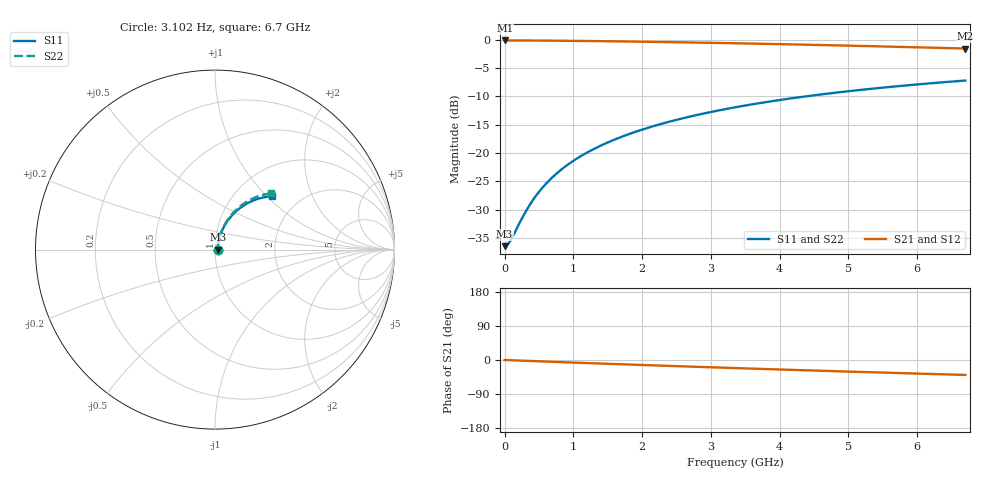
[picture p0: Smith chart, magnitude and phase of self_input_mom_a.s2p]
! Created Mon Jan 20 16:21:08 2014
# ghz S ma R 50
! 2 Port Network Data from data block
! freq  magS11  angS11  magS21  angS21  magS12  angS12  magS22  angS22
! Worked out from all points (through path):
!   107 points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, 3.102 Hz to 6.7 GHz, reference 50 ohm
!   highest |S21| = -0.13 dB at 3.102 MHz (marker M1); lowest = -1.6 dB at 6.7 GHz (marker M2)
!   group delay of S21, straight-line fit = 16.6 ps
!   lowest |S11| = -36.5 dB at 3.102 Hz (marker M3), VSWR 1.03, Z = 51.5 + j2.76e-08 ohm
!   |S11| at or under -10 dB: start of sweep to 4.386 GHz
!   |S22| runs from -36.5 to -7.1 dB; largest |S21 - S12| = 0
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3.101852e-09  0.01503 0.0  0.985 -0.0  0.985 -0.0  0.01503 0.0
0.003101852  0.01503 1.0  0.985 -0.0  0.985 -0.0  0.01503 1.0
0.03101852  0.01532 9.9  0.9849 -0.2  0.9849 -0.2  0.01529 9.9
0.06203704  0.01604 19.0  0.9849 -0.4  0.9849 -0.4  0.01602 19.0
0.09305556  0.01713 27.0  0.9848 -0.6  0.9848 -0.6  0.01712 27.1
0.2403935  0.02562 51.2  0.9843 -1.7  0.9843 -1.7  0.0256 51.3
0.3179398  0.03122 57.6  0.9839 -2.2  0.9839 -2.2  0.03118 57.7
0.4342593  0.04016 63.3  0.9831 -3.0  0.9831 -3.0  0.0401 63.4
0.5505787  0.04938 66.4  0.9821 -3.8  0.9821 -3.8  0.04932 66.6
0.6668981  0.05869 68.2  0.981 -4.6  0.981 -4.6  0.05865 68.5
0.7909722  0.06863 69.3  0.9796 -5.4  0.9796 -5.4  0.0686 69.6
0.9305556  0.07974 69.8  0.9779 -6.3  0.9779 -6.3  0.07973 70.3
1.116667  0.09439 70.0  0.9753 -7.5  0.9753 -7.5  0.09441 70.5
1.349306  0.1124 69.6  0.9717 -9.1  0.9717 -9.1  0.1124 70.2
1.628472  0.1334 68.7  0.967 -10.8  0.967 -10.8  0.1336 69.5
1.954167  0.1574 67.4  0.961 -12.9  0.961 -12.9  0.1576 68.3
2.303125  0.1823 65.8  0.954 -15.0  0.954 -15.0  0.1827 66.8
2.791667  0.216 63.3  0.9435 -18.0  0.9435 -18.0  0.2167 64.5
3.419792  0.2573 60.0  0.9286 -21.7  0.9286 -21.7  0.2585 61.4
4.466667  0.3209 54.4  0.9011 -27.6  0.9011 -27.6  0.3232 56.2
5.722917  0.3889 47.9  0.865 -34.4  0.865 -34.4  0.3929 50.0
6.7  0.436 43.0  0.8358 -39.4  0.8358 -39.4  0.4414 45.3
